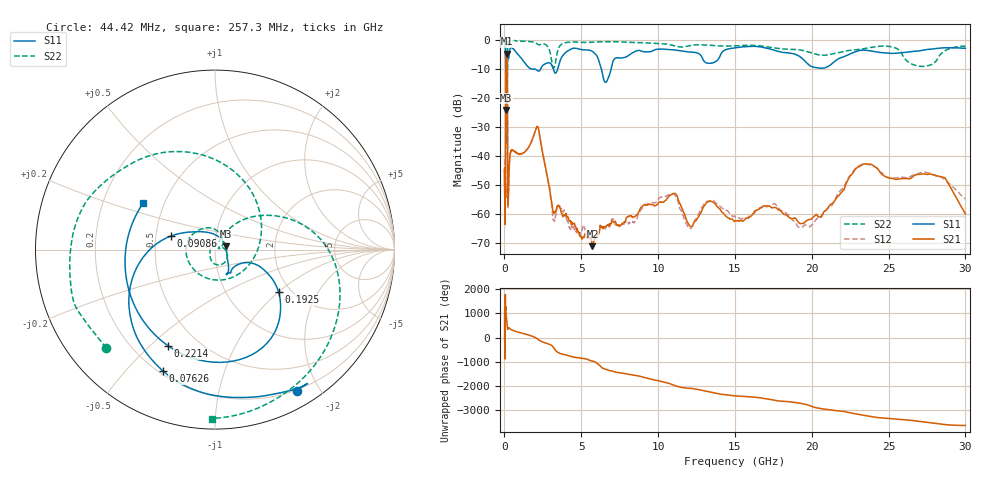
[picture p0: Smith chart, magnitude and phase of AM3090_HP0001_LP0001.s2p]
! Date/Time: Thu, Feb 28, 2019 1:53 PM
! Network Analyzer: Agilent Technologies E8364B Rev: A.07.50.67
! Sweep from 0.010 to 30.000 GHz, 1601 Points, Sweep Type: LOG
! Power Supply: 5.022 V, 0.002 A
# Hz S DB R 50
!freq MagS11 AngS11 MagS21 AngS21 MagS12 AngS12 MagS22 AngS22
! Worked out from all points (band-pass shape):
!   1601 points, 10 MHz to 30 GHz, reference 50 ohm
!   highest |S21| = -4.66 dB at 135.6 MHz (marker M1); lowest = -70.9 dB at 5.725 GHz (marker M2)
!   |S21| within 3 dB of the highest: 98.68 MHz to 177.5 MHz (78.85 MHz wide, 57.1 % of centre)
!   lowest |S11| = -24.1 dB at 98.44 MHz (marker M3), VSWR 1.13, Z = 56.4 + j2 ohm
!   |S11| at or under -10 dB: 1.991 GHz to 2.354 GHz (362.4 MHz wide, 16.7 % of centre); 3.182 GHz to 3.461 GHz (279.2 MHz wide, 8.41 % of centre); 6.309 GHz to 6.937 GHz (627.4 MHz wide, 9.47 % of centre)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
!   |S22| runs from -35.5 to -0.1 dB; largest |S21 - S12| = 0.013
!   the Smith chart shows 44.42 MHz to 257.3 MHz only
!   S11 on the Smith chart (normalised r, x): 44.42 MHz: 0.19, -1.72; 76.26 MHz: 0.22, -0.64; 90.86 MHz: 0.60, +0.10; 192.5 MHz: 1.73, -0.99; 221.4 MHz: 0.34, -0.57; 257.3 MHz: 0.38, +0.26
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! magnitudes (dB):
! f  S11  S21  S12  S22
! 10 MHz  -0.3  -44.8  -40.9  -0.5
! 38.04 MHz  -0.5  -60.7  -59.7  -1.4
! 44.42 MHz  -0.8  -57.6  -58.3  -1.8
! 76.26 MHz  -2.7  -42.8  -43.0  -5.1
! 90.86 MHz  -11.8  -14.0  -14.0  -15.5
! 98.44 MHz  -24.1  -7.8  -7.8  -16.2
! 135.6 MHz  -16.4  -4.7  -4.6  -28.0
! 144.7 MHz  -16.1  -4.8  -4.8  -21.7
! 170.7 MHz  -15.5  -6.4  -6.3  -33.1
! 192.5 MHz  -7.4  -17.7  -17.7  -10.4
! 221.4 MHz  -4.5  -55.7  -57.0  -1.4
! 257.3 MHz  -6.4  -52.6  -53.5  -0.5
! 550.5 MHz  -3.0  -37.9  -38.1  -0.2
! 2.084 GHz  -10.3  -30.1  -30.0  -1.2
! 3.204 GHz  -10.4  -59.7  -61.8  -9.6
! 5.725 GHz  -3.9  -70.9  -67.5  -0.8
! 6.619 GHz  -14.5  -64.2  -64.1  -0.6
! 7.926 GHz  -5.8  -61.3  -62.7  -0.7
! 10.7 GHz  -3.3  -53.8  -53.3  -1.5
! 19.7 GHz  -8.0  -62.0  -63.8  -4.0
! 23.48 GHz  -3.5  -42.6  -42.7  -2.9
! 30 GHz  -2.8  -59.8  -54.7  -2.1
